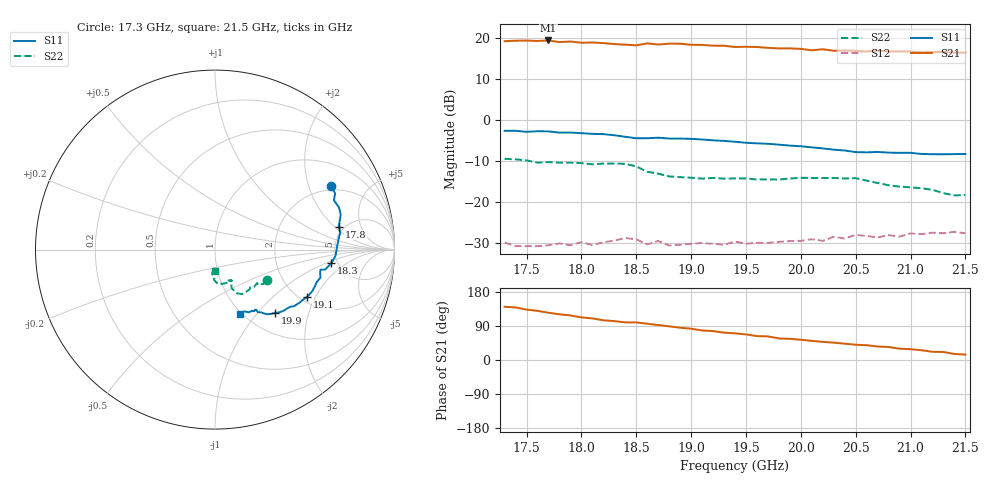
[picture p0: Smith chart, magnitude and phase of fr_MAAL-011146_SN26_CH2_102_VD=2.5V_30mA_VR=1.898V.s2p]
!Typical measured data - probed
!Date: Friday, August 19, 2022 11:47:41
!Correction: S11(Full 2 Port(1,2))
!S21(Full 2 Port(1,2))
!S12(Full 2 Port(1,2))
!S22(Full 2 Port(1,2))
!S2P File: Measurements: S11, S21, S12, S22:
# Hz S  dB  R 50
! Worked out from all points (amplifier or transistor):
!   43 points, 17.3 GHz to 21.5 GHz, reference 50 ohm
!   highest |S21| = 19.5 dB at 17.7 GHz (marker M1)
!   |S21| within 3 dB of that: start of sweep to end of sweep
!   unconditionally stable (mu >= 1): 17.45 GHz to 17.59 GHz; 17.71 GHz to end of sweep
!   at 18 GHz: K = 1.06, MAG = 22.9 dB, |S12| = -29.9 dB
!   at 19.4 GHz: K = 1.51, MAG = 19.6 dB, |S12| = -29.7 dB
!   at 21.5 GHz: K = 1.68, MAG = 17.3 dB, |S12| = -27.7 dB
!   S11 on the Smith chart (normalised r, x): 17.3 GHz: 1.84, +2.85; 17.8 GHz: 4.51, +2.27; 18.3 GHz: 4.43, -1.17; 19.1 GHz: 2.19, -1.73; 19.9 GHz: 1.35, -1.25; 21.5 GHz: 0.99, -0.83
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1.73e10  -2.64 28.5  19.31 140.5  -29.99 -35.8  -9.49 -30.8
1.74e10  -2.63 25.1  19.42 138.7  -30.87 -41.1  -9.62 -35.3
1.77e10  -2.78 15.4  19.49 124.7  -30.65 -36.0  -10.29 -39.0
1.78e10  -3.08 10.5  19.09 120.6  -30.21 -36.1  -10.45 -39.1
1.79e10  -3.05 7.8  19.23 117.5  -30.67 -39.8  -10.44 -43.5
1.8e10  -3.21 4.8  18.93 112.5  -29.89 -39.6  -10.54 -44.2
1.83e10  -3.71 -6.7  18.61 102.6  -29.52 -40.4  -10.67 -51.0
1.84e10  -4.10 -10.3  18.45 99.3  -28.89 -39.0  -10.71 -58.5
1.85e10  -4.46 -10.8  18.30 99.2  -29.20 -46.3  -11.35 -63.7
1.86e10  -4.45 -12.2  18.77 95.7  -30.44 -47.2  -12.66 -66.7
1.87e10  -4.32 -14.8  18.50 92.3  -29.60 -47.5  -13.13 -65.4
1.89e10  -4.54 -20.4  18.70 85.1  -30.53 -45.3  -13.98 -63.7
1.91e10  -4.76 -27.1  18.39 77.9  -30.12 -43.8  -14.34 -62.5
1.94e10  -5.32 -35.5  17.88 70.3  -29.75 -48.8  -14.28 -64.2
1.96e10  -5.70 -39.2  17.88 63.1  -30.05 -46.2  -14.56 -66.3
1.97e10  -5.81 -41.7  17.68 62.3  -30.07 -48.5  -14.52 -65.9
1.98e10  -6.03 -44.5  17.54 56.9  -29.82 -44.5  -14.58 -66.1
1.99e10  -6.25 -46.3  17.54 55.8  -29.64 -49.3  -14.32 -68.1
2.01e10  -6.69 -51.0  17.08 50.5  -29.18 -51.2  -14.18 -72.4
2.07e10  -7.81 -57.6  17.02 35.6  -28.76 -57.2  -15.41 -91.6
2.08e10  -7.97 -58.8  16.76 34.3  -28.19 -58.6  -15.97 -91.6
2.15e10  -8.31 -68.4  16.51 14.3  -27.73 -67.3  -18.34 -90.0
